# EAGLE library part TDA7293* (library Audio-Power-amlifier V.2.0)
120V - 100W DMOS Audio Amplifier with Mute/Standby
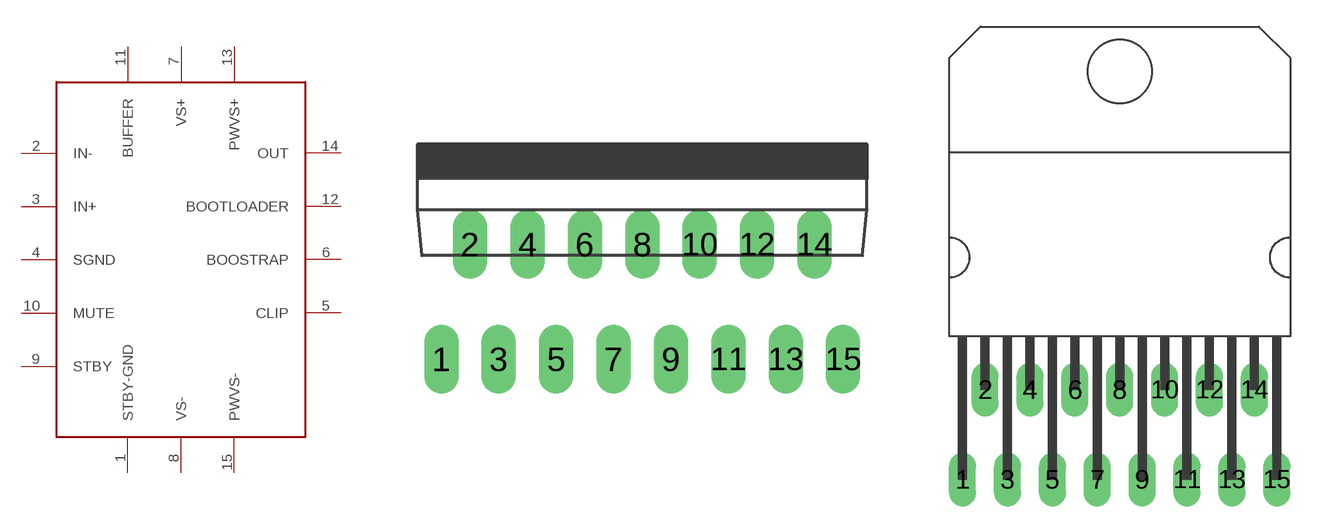
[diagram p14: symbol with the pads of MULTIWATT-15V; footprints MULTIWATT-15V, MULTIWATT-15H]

Designator prefix IC

## TDA7293VERTICAL  [MULTIWATT-15V]
1  STBY-GND  pwr
2  IN-  in
3  IN+  in
4  SGND  pwr
5  CLIP  oc
6  BOOSTRAP  pas
7  VS+  pwr
8  VS-  pwr
9  STBY  in
10  MUTE  in
11  BUFFER  pas
12  BOOTLOADER  pas
13  PWVS+  pwr
14  OUT  out
15  PWVS-  pwr

## TDA7293  [MULTIWATT-15H]
Pads as for MULTIWATT-15V

## Footprint MULTIWATT-15V (pad centres in mm)
Multiwatt 15 vertical
drill 1.016 long: 1 -8.89,-5.08; 2 -7.62,0; 3 -6.35,-5.08; 4 -5.08,0; 5 -3.81,-5.08; 6 -2.54,0; 7 -1.27,-5.08; 8 0,0; 9 1.27,-5.08; 10 2.54,0; 11 3.81,-5.08; 12 5.08,0; 13 6.35,-5.08; 14 7.62,0; 15 8.89,-5.08

## Footprint MULTIWATT-15H (pad centres in mm)
Multiwatt 15 horizontal
drill 1.016 long: 1 -8.89,-5.08; 2 -7.62,0; 3 -6.35,-5.08; 4 -5.08,0; 5 -3.81,-5.08; 6 -2.54,0; 7 -1.27,-5.08; 8 0,0; 9 1.27,-5.08; 10 2.54,0; 11 3.81,-5.08; 12 5.08,0; 13 6.35,-5.08; 14 7.62,0; 15 8.89,-5.08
